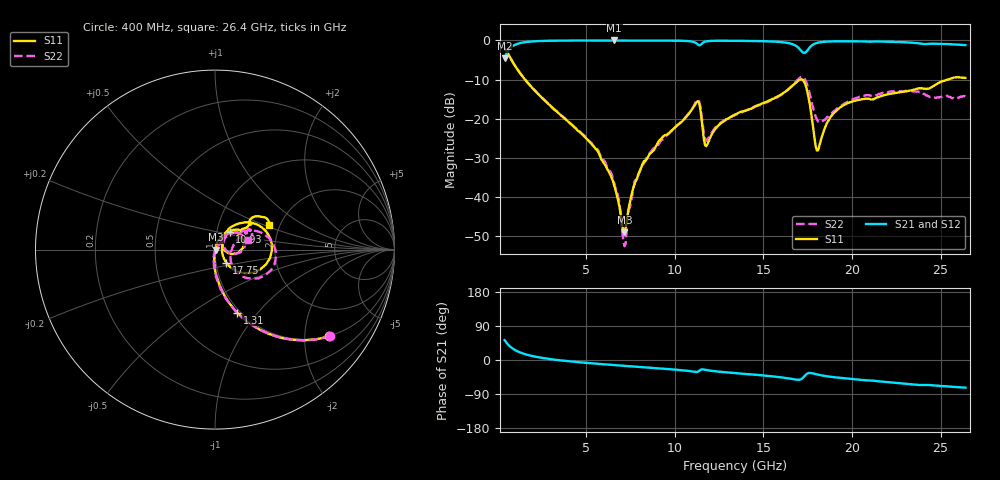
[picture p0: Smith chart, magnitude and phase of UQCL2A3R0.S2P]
! AVX Corporation
! Date:  10/27/06
! Part No:  UQCL2A3R0
! Description:  Ultra Low ESR Microwave capacitors
! Mounting Orientation:  Horizontal
# GHZ S DB R 50
! Freq  |S11|  S11 Ph  |S21|  S21 Ph  |S12|  S12 Ph  |S22|  S22 Ph
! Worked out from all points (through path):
!   401 points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, 400 MHz to 26.4 GHz, reference 50 ohm
!   highest |S21| = -0.03 dB at 6.575 GHz (marker M1); lowest = -4.5 dB at 400 MHz (marker M2)
!   group delay of S21, straight-line fit = 9.2 ps
!   lowest |S11| = -49.0 dB at 7.16 GHz (marker M3), VSWR 1.01, Z = 50.4 - j0.0404 ohm
!   |S11| at or under -10 dB: 1.551 GHz to 17.08 GHz (15.53 GHz wide, 167 % of centre); 17.18 GHz to 25.43 GHz (8.244 GHz wide, 38.7 % of centre)
!   |S22| runs from -52.5 to -1.9 dB; largest |S21 - S12| = 0.0049
!   S11 on the Smith chart (normalised r, x): 400 MHz: 0.99, -2.63; 1.31 GHz: 0.97, -0.79; 10.93 GHz: 1.16, +0.23; 17.75 GHz: 1.12, -0.16; 26.4 GHz: 1.77, +0.54
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0.4  -1.96 -37.3  -4.53 52.2  -4.50 52.2  -1.92 -37.1
0.855  -5.55 -59.5  -1.46 30.2  -1.44 30.2  -5.51 -59.3
1.31  -8.60 -70.6  -0.66 19.3  -0.64 19.2  -8.57 -70.6
4.755  -23.83 -93.5  -0.04 -6.5  -0.03 -6.7  -23.81 -97.0
5.6  -27.91 -95.8  -0.05 -9.9  -0.04 -10.0  -27.66 -101.0
6.575  -36.80 -86.3  -0.03 -13.4  -0.03 -13.6  -36.33 -97.2
7.16  -48.96 -6.5  -0.03 -15.4  -0.04 -15.6  -52.47 -49.5
7.81  -35.77 62.2  -0.03 -17.7  -0.04 -17.9  -35.25 57.9
9.11  -25.63 71.7  -0.06 -22.2  -0.08 -22.4  -26.39 52.8
10.93  -17.88 49.8  -0.28 -29.8  -0.28 -29.9  -17.75 47.7
11.32  -15.52 16.4  -1.13 -30.5  -1.14 -30.6  -15.16 16.4
11.775  -26.99 23.1  -0.28 -26.4  -0.28 -26.5  -25.58 15.6
13.4  -18.94 57.9  -0.11 -34.5  -0.12 -34.5  -19.07 46.8
16.39  -12.56 40.2  -0.68 -48.3  -0.70 -48.3  -12.58 27.0
17.105  -9.95 5.6  -2.50 -51.2  -2.52 -51.1  -9.38 -1.8
17.43  -12.16 -31.4  -2.88 -37.3  -2.90 -37.2  -10.73 -33.4
17.755  -20.41 -49.2  -1.23 -35.1  -1.25 -35.0  -16.33 -45.8
18.08  -28.07 11.7  -0.60 -38.8  -0.62 -38.7  -20.68 -22.1
18.665  -20.49 52.2  -0.30 -43.4  -0.32 -43.3  -19.42 14.2
19.315  -17.18 49.2  -0.24 -47.1  -0.26 -47.0  -16.86 25.4
22.11  -13.66 35.3  -0.38 -58.7  -0.40 -58.5  -13.09 31.1
26.4  -9.58 24.0  -1.21 -73.0  -1.22 -72.7  -14.30 15.5
